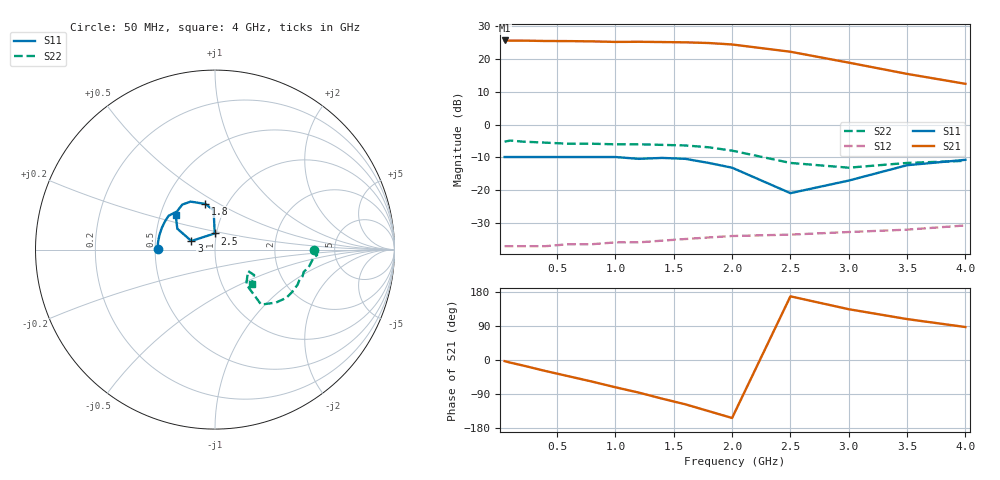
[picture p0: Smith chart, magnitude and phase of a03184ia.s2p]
!  INA-03184  S PARAMETERS
!  Id = 10 mA  LAST UPDATED 07-22-92
# ghz s ma r 50
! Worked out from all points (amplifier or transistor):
!   16 points, 50 MHz to 4 GHz, reference 50 ohm
!   highest |S21| = 25.6 dB at 50 MHz (marker M1)
!   |S21| within 3 dB of that: start of sweep to 2.401 GHz
!   unconditionally stable (mu >= 1): start of sweep to end of sweep
!   at 200 MHz: K = 1.48, MAG = 27.2 dB, |S12| = -37.1 dB
!   at 1.4 GHz: K = 1.42, MAG = 26.4 dB, |S12| = -35.4 dB
!   at 4 GHz: K = 3.52, MAG = 13.2 dB, |S12| = -30.8 dB
!   S11 on the Smith chart (normalised r, x): 50 MHz: 0.52, +0.01; 1.8 GHz: 0.79, +0.43; 2.5 GHz: 0.98, +0.18; 3 GHz: 0.76, +0.07; 4 GHz: 0.60, +0.25
0.05  0.32 179.0  19.14 -3.0  0.014 3.0  0.55 0.0
0.1  0.32 176.0  19.05 -7.0  0.014 4.0  0.57 -3.0
0.2  0.32 172.0  19.05 -14.0  0.014 6.0  0.55 -5.0
0.4  0.32 165.0  18.78 -29.0  0.014 10.0  0.53 -11.0
0.6  0.32 158.0  18.71 -43.0  0.015 11.0  0.51 -14.0
0.8  0.32 151.0  18.53 -57.0  0.015 13.0  0.51 -17.0
1  0.32 144.0  18.18 -72.0  0.016 21.0  0.5 -20.0
1.2  0.3 135.0  18.27 -86.0  0.016 25.0  0.5 -23.0
1.4  0.31 126.0  18.1 -102.0  0.017 30.0  0.49 -29.0
1.6  0.3 117.0  17.92 -117.0  0.018 38.0  0.48 -34.0
1.8  0.26 102.0  17.49 -135.0  0.019 44.0  0.45 -41.0
2  0.22 92.0  16.62 -153.0  0.02 49.0  0.4 -50.0
2.5  0.09 91.0  12.88 168.0  0.021 57.0  0.26 -48.0
3  0.14 160.0  8.79 134.0  0.023 65.0  0.22 -33.0
3.5  0.24 151.0  5.92 108.0  0.025 69.0  0.26 -33.0
4  0.29 139.0  4.18 87.0  0.029 81.0  0.28 -43.0
